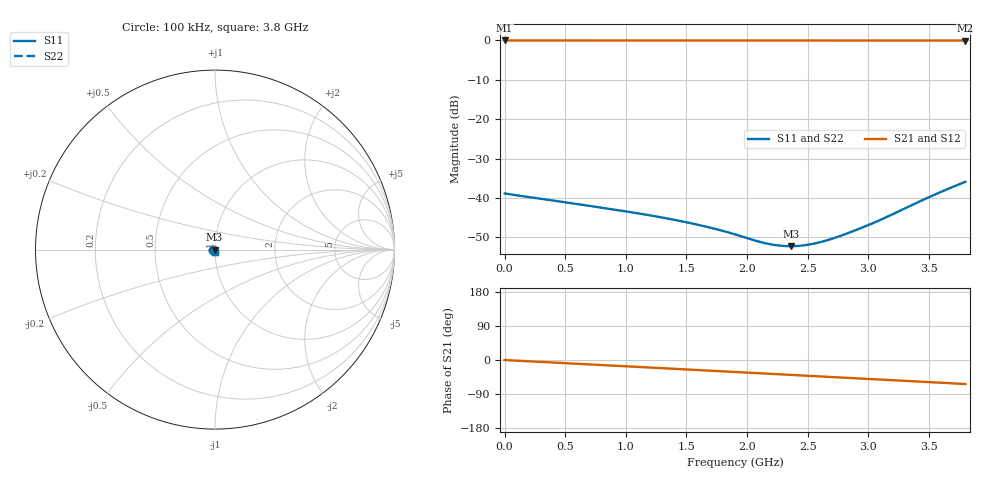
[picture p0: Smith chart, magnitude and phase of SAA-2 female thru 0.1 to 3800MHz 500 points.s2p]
! ListType=Lin
!!SAA-2 female thru 0.1 to 3800MHz 500 points
# MHZ S RI R 50
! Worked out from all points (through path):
!   500 points, 100 kHz to 3.8 GHz, reference 50 ohm
!   highest |S21| = 0.00 dB at 100 kHz (marker M1); lowest = 0.0 dB at 3.8 GHz (marker M2)
!   group delay of S21, straight-line fit = 46.2 ps
!   lowest |S11| = -52.3 dB at 2.361 GHz (marker M3), VSWR 1.00, Z = 49.8 - j0.0346 ohm
!   |S11| at or under -10 dB: start of sweep to end of sweep
!   |S22| runs from -52.3 to -35.9 dB; largest |S21 - S12| = 0
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0.1  -0.0114 -0.000356  0.9999 -0.00141  0.9999 -0.00141  -0.0114 -0.000356
312.3162  -0.00933 0.00258  0.9951 -0.0908  0.9951 -0.0908  -0.00933 0.00258
639.7625  -0.00762 0.00296  0.9815 -0.1842  0.9815 -0.1842  -0.00762 0.00296
951.9788  -0.00578 0.0038  0.9606 -0.2719  0.9606 -0.2719  -0.00578 0.0038
1271.81  -0.00405 0.00407  0.9313 -0.3596  0.9313 -0.3596  -0.00405 0.00407
1446.956  -0.00354 0.00366  0.9119 -0.4063  0.9119 -0.4063  -0.00354 0.00366
1614.486  -0.00328 0.00306  0.8912 -0.4501  0.8912 -0.4501  -0.00328 0.00306
1766.787  -0.00314 0.00237  0.8706 -0.489  0.8706 -0.489  -0.00314 0.00237
1903.858  -0.003 0.00167  0.8505 -0.5232  0.8505 -0.5232  -0.003 0.00167
2063.773  -0.00275 0.000831  0.8255 -0.5621  0.8255 -0.5621  -0.00275 0.000831
2162.769  -0.0026 0.000396  0.8091 -0.5856  0.8091 -0.5856  -0.0026 0.000396
2261.764  -0.00248 1.42e-05  0.7921 -0.6086  0.7921 -0.6086  -0.00248 1.42e-05
2360.759  -0.00241 -0.000347  0.7744 -0.6311  0.7744 -0.6311  -0.00241 -0.000347
2444.525  -0.00239 -0.000664  0.7589 -0.6497  0.7589 -0.6497  -0.00239 -0.000664
2535.905  -0.00238 -0.00105  0.7415 -0.6696  0.7415 -0.6696  -0.00238 -0.00105
2657.745  -0.00237 -0.00165  0.7174 -0.6954  0.7174 -0.6954  -0.00237 -0.00165
2794.816  -0.00228 -0.00252  0.6893 -0.7234  0.6893 -0.7234  -0.00228 -0.00252
3015.652  -0.00163 -0.00433  0.6417 -0.766  0.6417 -0.766  -0.00163 -0.00433
3167.953  -0.000827 -0.00583  0.6071 -0.7937  0.6071 -0.7937  -0.000827 -0.00583
3541.089  0.000879 -0.0109  0.5151 -0.8554  0.5151 -0.8554  0.000879 -0.0109
3708.62  0.00048 -0.0141  0.4708 -0.8799  0.4708 -0.8799  0.00048 -0.0141
3800  -0.000469 -0.016  0.4459 -0.8923  0.4459 -0.8923  -0.000469 -0.016
